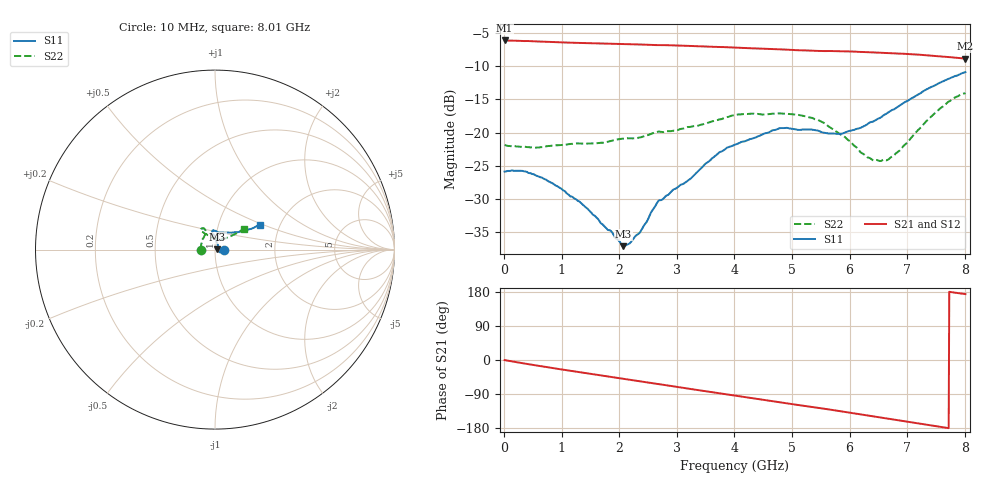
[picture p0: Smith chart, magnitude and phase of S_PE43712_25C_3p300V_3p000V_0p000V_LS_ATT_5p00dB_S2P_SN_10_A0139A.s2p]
! DEVICE ID: PE43712
! File Path: z:\PE43713\PE43713_CHAR_NOM_04292014\AMB\3p300\LS_ATT_5p00dB\PE43713_AMB_3p300V_3p000V_0p000V_LS_ATT_5p00dB_S2P_SN_10_A0139A.s2p
! Serial: 10
! Lot: A0139A
! Temp: 25C
! VDD: 3.300
! VSS: 0.000
! Control_Hi: 3.000
! Control_Lo: 0.000
! Attenuation Step: 5.00dB
! Port 1: RF1
! Port 2: RF2
! ThroughPath:1-2
! IDD: 0.0001471956
! ISS: -1.071e-007
#  Hz  S  RI  R  50
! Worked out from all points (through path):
!   801 points, 10 MHz to 8.01 GHz, reference 50 ohm
!   highest |S21| = -6.11 dB at 10 MHz (marker M1); lowest = -8.8 dB at 8.01 GHz (marker M2)
!   group delay of S21, straight-line fit = 63.9 ps
!   lowest |S11| = -37.1 dB at 2.07 GHz (marker M3), VSWR 1.03, Z = 51.4 + j0.0929 ohm
!   |S11| at or under -10 dB: start of sweep to end of sweep
!   |S22| runs from -24.3 to -14.1 dB; largest |S21 - S12| = 0.0015
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1e7  0.0507 -0.000106  0.4947 -0.00283  0.4945 -0.00273  -0.0805 0.000491
3.4e8  0.0502 -0.00974  0.4841 -0.0758  0.4839 -0.0746  -0.0777 0.00652
6.3e8  0.0437 -0.0146  0.4666 -0.1343  0.4666 -0.1344  -0.0764 0.0127
9.6e8  0.0348 -0.0164  0.4382 -0.195  0.4384 -0.195  -0.0777 0.0206
1.35e9  0.0251 -0.0144  0.3972 -0.2578  0.3972 -0.2578  -0.0767 0.0306
2.07e9  0.0139 0.000903  0.3017 -0.3536  0.3018 -0.3534  -0.0707 0.0557
2.18e9  0.014 0.00398  0.2852 -0.3656  0.2852 -0.3654  -0.0684 0.0592
2.36e9  0.0137 0.0111  0.2562 -0.3836  0.2563 -0.3835  -0.0628 0.067
2.68e9  0.0162 0.0259  0.2037 -0.4084  0.2038 -0.4084  -0.0534 0.0865
3.23e9  0.00814 0.0438  0.1066 -0.4368  0.1067 -0.4369  -0.0518 0.0973
3.72e9  0.00269 0.0698  0.0198 -0.4415  0.0196 -0.4414  -0.0555 0.1119
4.01e9  -0.0041 0.081  -0.0316 -0.4364  -0.0315 -0.4363  -0.0653 0.1188
4.79e9  -0.0135 0.1071  -0.1572 -0.3938  -0.1573 -0.3941  -0.0784 0.1152
5.35e9  -0.00112 0.1051  -0.2326 -0.3431  -0.2325 -0.3428  -0.077 0.1034
5.55e9  0.00951 0.0993  -0.2559 -0.3223  -0.2557 -0.3223  -0.0674 0.0974
5.87e9  0.0266 0.0945  -0.2948 -0.2858  -0.2943 -0.2859  -0.045 0.0839
6.38e9  0.0728 0.0956  -0.3404 -0.2145  -0.3399 -0.2143  -0.00349 0.0628
6.68e9  0.1059 0.0959  -0.3596 -0.1681  -0.3593 -0.1681  0.0257 0.0576
6.87e9  0.1263 0.0972  -0.3689 -0.1381  -0.3685 -0.138  0.043 0.0593
7.55e9  0.2045 0.1168  -0.3746 -0.027  -0.3742 -0.0271  0.1184 0.0903
7.81e9  0.2302 0.1302  -0.3677 0.0115  -0.3675 0.0113  0.1468 0.1073
8.01e9  0.2495 0.1394  -0.359 0.0381  -0.3584 0.0376  0.1605 0.1164
